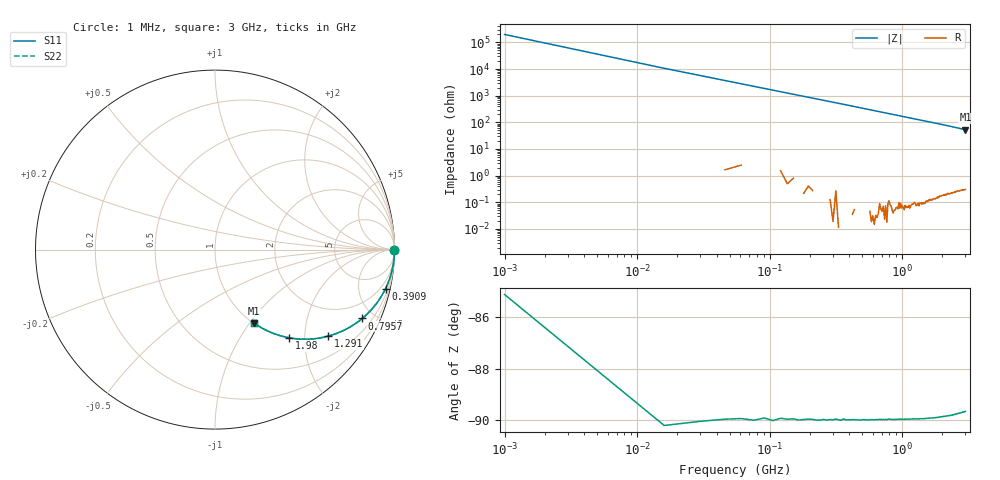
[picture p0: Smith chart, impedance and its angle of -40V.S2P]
!Keysight Technologies,E4991B,MY54301043,A.02.04
!Date: Thu Nov 16 21:17:35 2023
!Data:
!Freq	S11	S21	S12	S22
# Hz S MA R 50
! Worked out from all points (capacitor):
!   201 points, 1 MHz to 3 GHz, reference 50 ohm
!   read as one part in series: C = 931 fF near 15.99 MHz
!   lowest |Z| = 52.7 ohm at 3 GHz (marker M1)
!   S11 on the Smith chart (normalised r, x): 1 MHz: open; 390.9 MHz: 1.00, -8.74; 795.7 MHz: 1.00, -4.28; 1.291 GHz: 1.00, -2.62; 1.98 GHz: 1.00, -1.68; 3 GHz: 1.01, -1.05
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1000000  1 -0.0  0.0005052 85.1  0.0005052 85.1  1 -0.0
1.5995e7  1 -0.5  0.009377 89.7  0.009377 89.7  1 -0.5
3.099e7  0.9999 -1.0  0.01812 89.0  0.01812 89.0  0.9999 -1.0
4.5985e7  0.9996 -1.5  0.02689 88.4  0.02689 88.4  0.9996 -1.5
6.098e7  0.9993 -2.0  0.03561 87.9  0.03561 87.9  0.9993 -2.0
7.5975e7  0.999 -2.5  0.04437 87.5  0.04437 87.5  0.999 -2.5
1.05965e8  0.9981 -3.5  0.06184 86.5  0.06184 86.5  0.9981 -3.5
1.35955e8  0.9968 -4.5  0.07929 85.4  0.07929 85.4  0.9968 -4.5
1.8094e8  0.9944 -6.0  0.1052 83.9  0.1052 83.9  0.9944 -6.0
2.25925e8  0.9914 -7.5  0.131 82.5  0.131 82.5  0.9914 -7.5
2.7091e8  0.9877 -9.0  0.1565 81.0  0.1565 81.0  0.9877 -9.0
3.9087e8  0.9748 -12.9  0.223 77.1  0.223 77.1  0.9748 -12.9
5.1083e8  0.958 -16.7  0.2866 73.3  0.2866 73.3  0.958 -16.7
6.45785e8  0.9352 -20.7  0.3541 69.3  0.3541 69.3  0.9352 -20.7
7.95735e8  0.9058 -25.0  0.4232 64.9  0.4232 64.9  0.9058 -25.0
1.005665e9  0.8604 -30.6  0.5093 59.4  0.5093 59.4  0.8604 -30.6
1.29057e9  0.7948 -37.3  0.6064 52.6  0.6064 52.6  0.7948 -37.3
1.5005e9  0.7464 -41.7  0.6648 48.3  0.6648 48.3  0.7464 -41.7
1.98034e9  0.6424 -49.9  0.765 40.0  0.765 40.0  0.6424 -49.9
2.01033e9  0.6364 -50.4  0.77 39.5  0.77 39.5  0.6364 -50.4
2.505165e9  0.5438 -56.8  0.8371 32.9  0.8371 32.9  0.5438 -56.8
3e9  0.4648 -62.0  0.8827 27.7  0.8827 27.7  0.4648 -62.0
